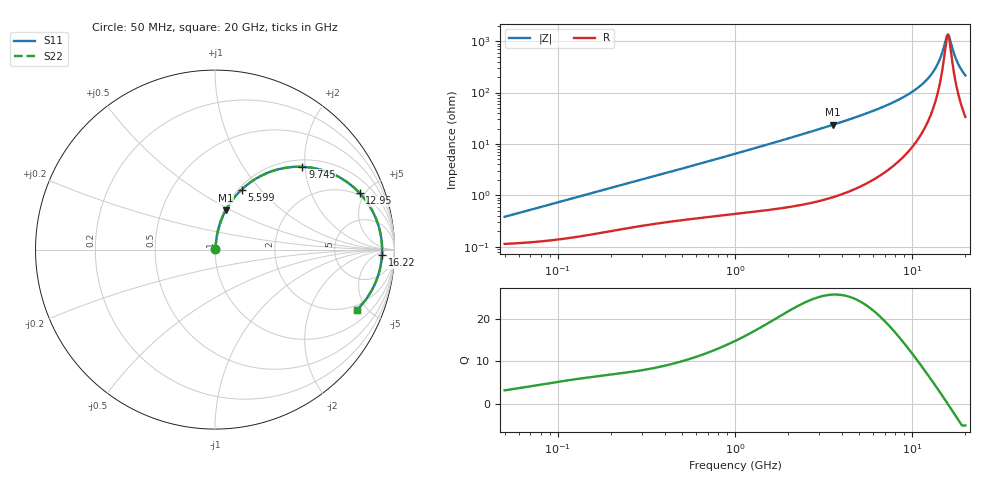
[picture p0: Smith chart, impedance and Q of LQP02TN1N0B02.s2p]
!Murata Part Number: LQP02TN1N0B02
!These Parameters are Measured in Series Mode Connection
!  o--[Z]--o
!Port1  Port2
!  o-------o
!Freq. Start=50[MHz] Stop=20[GHz], 401[Steps]
# Hz S RI R 50
!Freq.(Hz) S11(Real) S11(Imag) S21(Real) S21(Imag) S12(Real) S12(Imag) S22(Real) S22(Imag)
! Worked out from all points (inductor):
!   401 points, 50 MHz to 20 GHz, reference 50 ohm
!   read as one part in series: L = 1.16 nH near 51.52 MHz
!   highest Q = 25.6 at 3.572 GHz (marker M1), where L = 1.05 nH
!   self-resonance near 15.93 GHz
!   S11 on the Smith chart (normalised r, x): 50 MHz: 1.00, +0.01; 5.599 GHz: 1.03, +0.80; 9.745 GHz: 1.16, +1.94; 12.95 GHz: 1.85, +4.63; 16.22 GHz: 23, -10; 20 GHz: 1.67, -4.26
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5e7  0.00115 0.00365  0.9989 -0.00365  0.9989 -0.00365  0.00115 0.00365
1.364002e8  0.0017 0.0097  0.9983 -0.0097  0.9983 -0.0097  0.0017 0.0097
3.721004e8  0.00347 0.0248  0.9965 -0.0248  0.9965 -0.0248  0.00347 0.0248
1e9  0.00839 0.0634  0.9916 -0.0634  0.9916 -0.0634  0.00839 0.0634
2.728004e9  0.0368 0.169  0.9632 -0.169  0.9632 -0.169  0.0368 0.169
3.572216e9  0.0605 0.2197  0.9395 -0.2197  0.9395 -0.2197  0.0605 0.2197
5.598765e9  0.1487 0.3347  0.8513 -0.3347  0.8513 -0.3347  0.1487 0.3347
7.442007e9  0.2729 0.419  0.7271 -0.419  0.7271 -0.419  0.2729 0.419
9.745021e9  0.4871 0.4613  0.5129 -0.4613  0.5129 -0.4613  0.4871 0.4613
1.149051e10  0.6708 0.4147  0.3292 -0.4147  0.3292 -0.4147  0.6708 0.4147
1.295331e10  0.8072 0.3135  0.1928 -0.3135  0.1928 -0.3135  0.8072 0.3135
1.354865e10  0.8511 0.2583  0.1489 -0.2583  0.1489 -0.2583  0.8511 0.2583
1.417136e10  0.8874 0.1945  0.1126 -0.1945  0.1126 -0.1945  0.8874 0.1945
1.460232e10  0.9062 0.1479  0.0938 -0.1479  0.0938 -0.1479  0.9062 0.1479
1.550395e10  0.9285 0.0477  0.0715 -0.0477  0.0715 -0.0477  0.9285 0.0477
1.573793e10  0.9305 0.0218  0.0695 -0.0218  0.0695 -0.0218  0.9305 0.0218
1.597544e10  0.9312 -0.00414  0.0688 0.00414  0.0688 0.00414  0.9312 -0.00414
1.621653e10  0.9303 -0.0301  0.0697 0.0301  0.0697 0.0301  0.9303 -0.0301
1.747767e10  0.905 -0.156  0.095 0.156  0.095 0.156  0.905 -0.156
1.800918e10  0.8858 -0.2026  0.1142 0.2026  0.1142 0.2026  0.8858 -0.2026
1.912117e10  0.8348 -0.2855  0.1652 0.2855  0.1652 0.2855  0.8348 -0.2855
2e10  0.7884 -0.3373  0.2116 0.3373  0.2116 0.3373  0.7884 -0.3373
